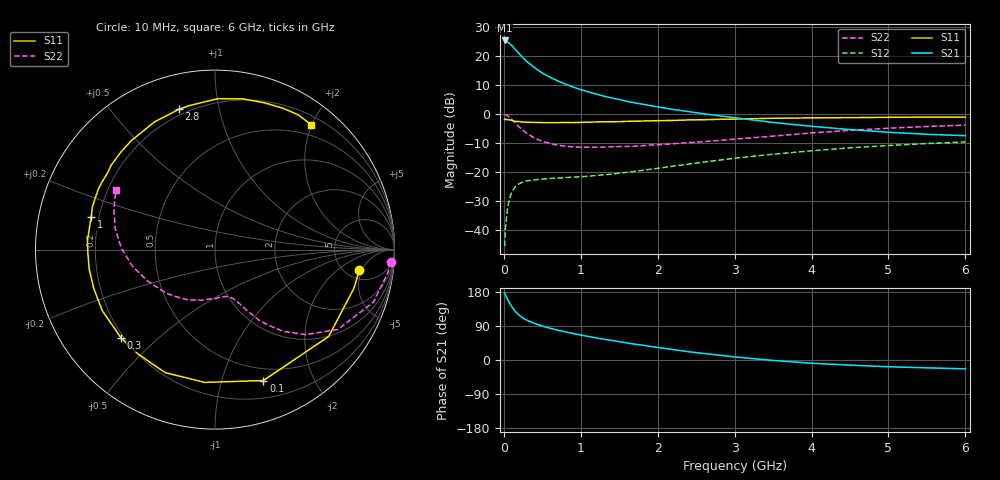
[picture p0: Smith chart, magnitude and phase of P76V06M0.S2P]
! SIEMENS Small Signal Semiconductors
! BFP196
! Si NPN RF Bipolar Junction Transistor in SOT143
! VCE = 6 V  IC = 6 mA
! Common Emitter S-Parameters:  May  1996
# GHz  S  MA  R  50
!  f  S11  S21  S12  S22
! GHz  MAG  ANG  MAG  ANG  MAG  ANG  MAG  ANG
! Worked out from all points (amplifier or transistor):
!   36 points, 10 MHz to 6 GHz, reference 50 ohm
!   highest |S21| = 25.3 dB at 10 MHz (marker M1)
!   |S21| within 3 dB of that: start of sweep to 144.6 MHz
!   unconditionally stable (mu >= 1): 1.091 GHz to 3.198 GHz
!   at 250 MHz: K = 0.28, MSG = 21.3 dB, |S12| = -23.4 dB
!   at 1.4 GHz: K = 1.14, MAG = 10.8 dB, |S12| = -20.7 dB
!   at 6 GHz: K = 0.98, MSG = 1.1 dB, |S12| = -9.6 dB
!   S11 on the Smith chart (normalised r, x): 10 MHz: 6.62, -4.46; 100 MHz: 0.37, -1.37; 300 MHz: 0.19, -0.39; 1 GHz: 0.17, +0.13; 2.8 GHz: 0.17, +0.76; 6 GHz: 0.33, +1.99
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0.01  0.8127 -8.1  18.37 176.6  0.0053 86.6  0.9832 -3.9
0.02  0.8034 -15.6  18.04 171.0  0.0104 81.0  0.9725 -7.5
0.05  0.7972 -37.4  17.37 159.2  0.0256 71.4  0.9308 -18.3
0.1  0.7777 -69.7  15.18 141.8  0.045 56.8  0.8155 -33.1
0.15  0.7422 -94.4  12.76 128.0  0.0563 46.1  0.6932 -43.1
0.2  0.7396 -112.1  10.84 118.3  0.0628 39.1  0.5953 -50.0
0.25  0.7225 -126.2  9.167 110.7  0.0677 34.0  0.5187 -54.6
0.3  0.7185 -136.6  7.964 105.0  0.0704 31.0  0.4628 -58.1
0.4  0.7144 -151.6  6.239 96.5  0.0733 27.2  0.3831 -62.3
0.5  0.7092 -162.2  5.054 89.6  0.0754 25.4  0.3372 -65.1
0.6  0.7094 -171.0  4.277 83.8  0.0774 25.0  0.3096 -67.4
0.7  0.7085 -178.3  3.708 78.6  0.0785 25.2  0.2906 -69.9
0.8  0.7123 175.9  3.256 74.2  0.0802 25.7  0.2783 -72.4
1  0.7135 165.2  2.617 65.9  0.0829 27.9  0.2678 -77.1
1.1  0.7235 160.7  2.392 62.1  0.0847 29.3  0.2674 -79.8
1.6  0.7453 141.0  1.647 45.1  0.099 35.8  0.2761 -94.9
2.2  0.7717 121.6  1.195 27.5  0.1262 40.1  0.3066 -113.4
2.8  0.8075 104.4  0.93 12.7  0.16 39.1  0.35 -133.2
3.5  0.8411 88.9  0.713 -1.2  0.2025 33.6  0.4146 -155.1
4.5  0.863 71.4  0.538 -13.6  0.2608 22.8  0.5217 179.1
5.5  0.8826 58.3  0.446 -20.7  0.3089 10.6  0.6074 158.1
6  0.8786 52.4  0.422 -23.3  0.3305 4.2  0.6429 149.1
